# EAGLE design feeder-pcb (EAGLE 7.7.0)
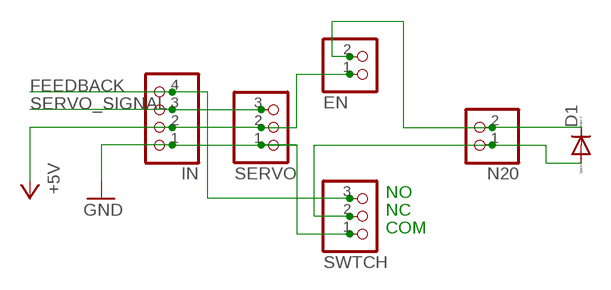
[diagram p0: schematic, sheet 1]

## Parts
D1  DIODE-D-7.5  [D-7.5]
EN  PINHD-1X2  [1X02]
IN  PINHD-1X4  [1X04]
N20  PINHD-1X2  [1X02]
SERVO  PINHD-1X3  [1X03]
SWTCH  PINHD-1X3  [1X03]

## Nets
+5V: EN.1 IN.2 SERVO.2
FEEDBACK: IN.4 SWTCH.3
GND: IN.1 SERVO.1 SWTCH.1
N$1: D1.A N20.1 SWTCH.2
N$2: D1.C EN.2 N20.2
SERVO_SIGNAL: IN.3 SERVO.3

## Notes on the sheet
- NO
- NC
- COM

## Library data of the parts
D1 = diode:DIODE-: DIODE
EN N20 = pinhead:PINHD-1X2: PIN HEADER
IN = pinhead:PINHD-1X4: PIN HEADER
SERVO SWTCH = pinhead:PINHD-1X3: PIN HEADER

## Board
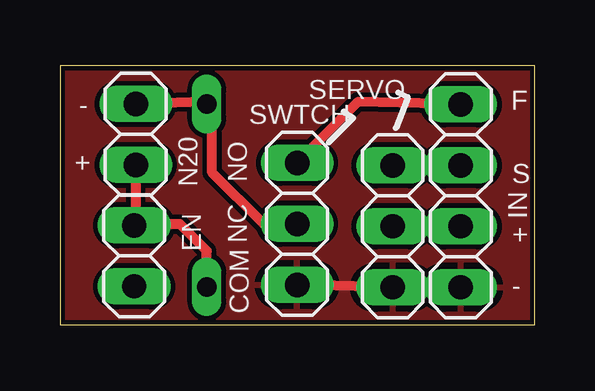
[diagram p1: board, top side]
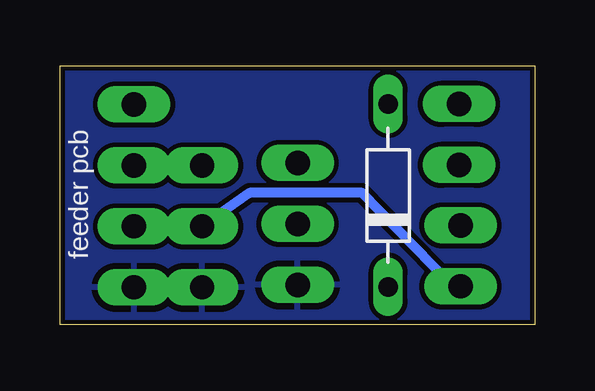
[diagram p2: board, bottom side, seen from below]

Size 19.8 x 10.8 mm. Coordinates in mm from the lower left corner, seen from the top.
Outline: 0,0 19.8,0 19.8,10.8 0,10.8 0,0
Copper layers (1*16): Top 0.0356mm / dielectric 1.5011mm / Bottom 0.0356mm
Design rules "oshpark-2layer *": minimum track width 6mil, minimum drill 13mil, track to track 6mil, track to pad 6mil, pad to pad 6mil, via to via 6mil, smd to smd 6mil, copper to edge 0.2mm, drill to drill 6mil, minimum pad ring 7mil, minimum via ring 7mil, stop-mask expansion 2.5mil, vias tented up to drill 0mil, thermal gap 10mil

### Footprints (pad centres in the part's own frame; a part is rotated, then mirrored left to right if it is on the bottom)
D-7.5 = drill 0.813 long: A 3.81,0; C -3.81,0
1X02 = drill 1.016 long: 1 -1.27,0; 2 1.27,0
1X04 = drill 1.016 long: 1 -3.81,0; 2 -1.27,0; 3 1.27,0; 4 3.81,0
1X03 = drill 1.016 long: 1 -2.54,0; 2 0,0; 3 2.54,0

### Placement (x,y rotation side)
D1  6.12,5.4 90 bottom
EN  3.1,2.88 90 top
IN  16.71,5.38 90 top
N20  3.16,7.94 270 top
SERVO  13.88,4.11 90 top
SWTCH  9.89,4.21 90 top

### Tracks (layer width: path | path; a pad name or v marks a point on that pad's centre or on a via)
+5V
  Top 0.406: IN.2 SERVO.2
  Bottom 0.406: EN.1 3.51,1.71 7.2,5.5 11.88,5.5 SERVO.2
FEEDBACK
  Top 0.406: IN.4 12.43,9.29 SWTCH.3
GND
  Top 0.406: IN.1 SERVO.1 SWTCH.1
  pour Top (isolate 0.2): 0,12 22,12 22,0 0,0
  pour Bottom (isolate 0.2): 0,12 22,12 22,0 0,0
N$1
  Top 0.406: N20.1 6.01,9.31 D1.A 6.35,8.97 6.35,6.35 8.49,4.21 SWTCH.2
N$2
  Top 0.406: D1.C 6.12,3.08 5,4.2 3.15,4.2 EN.2 3.16,4.32 N20.2
SERVO_SIGNAL
  Top 0.406: IN.3 SERVO.3

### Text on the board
tPlace: - | F | + | NO | S | NC | + | - | COM
bPlace: feeder pcb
